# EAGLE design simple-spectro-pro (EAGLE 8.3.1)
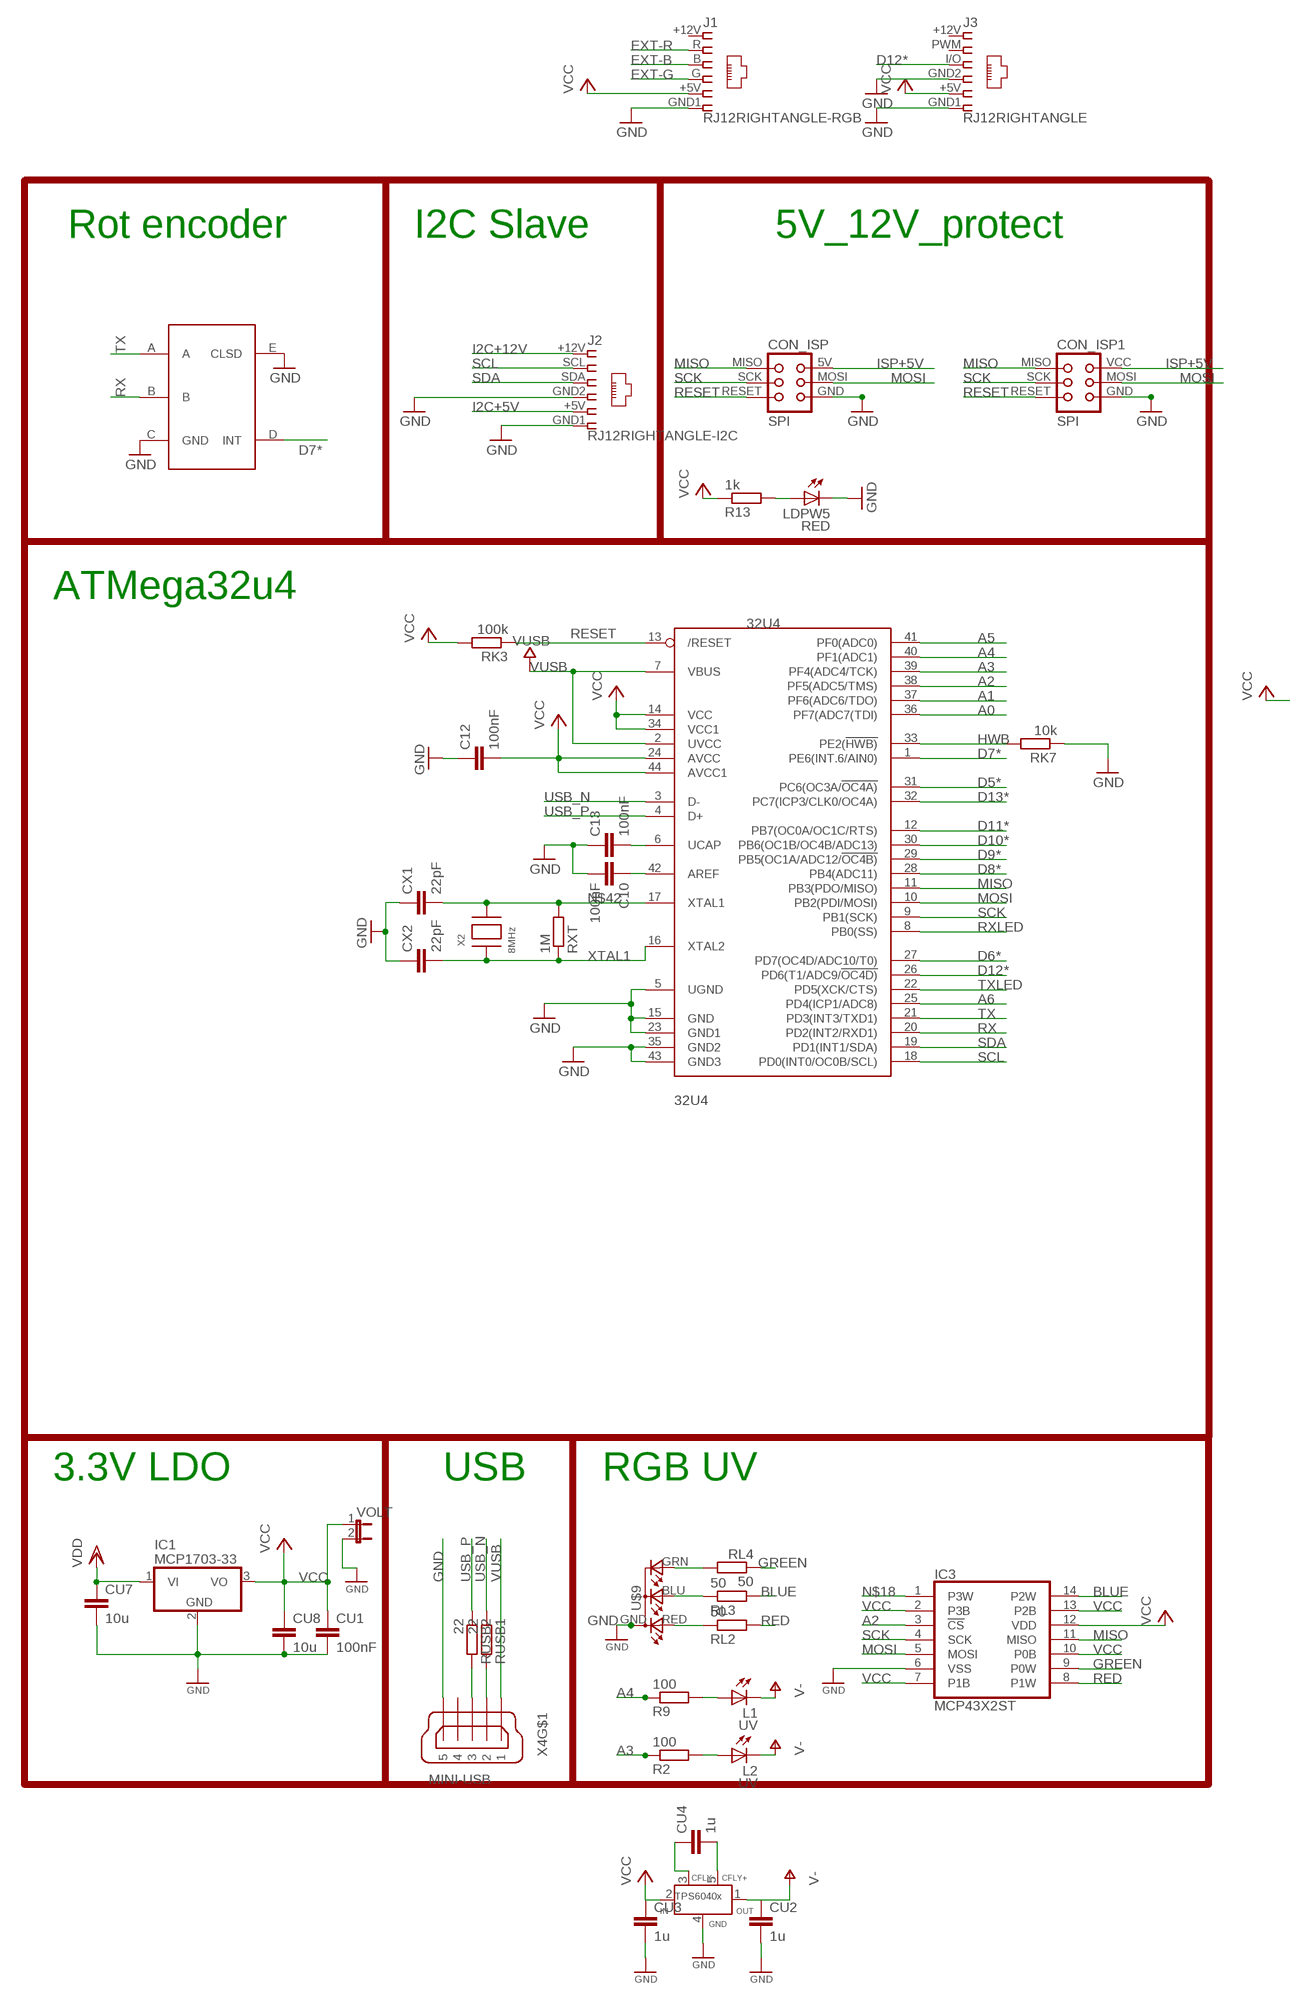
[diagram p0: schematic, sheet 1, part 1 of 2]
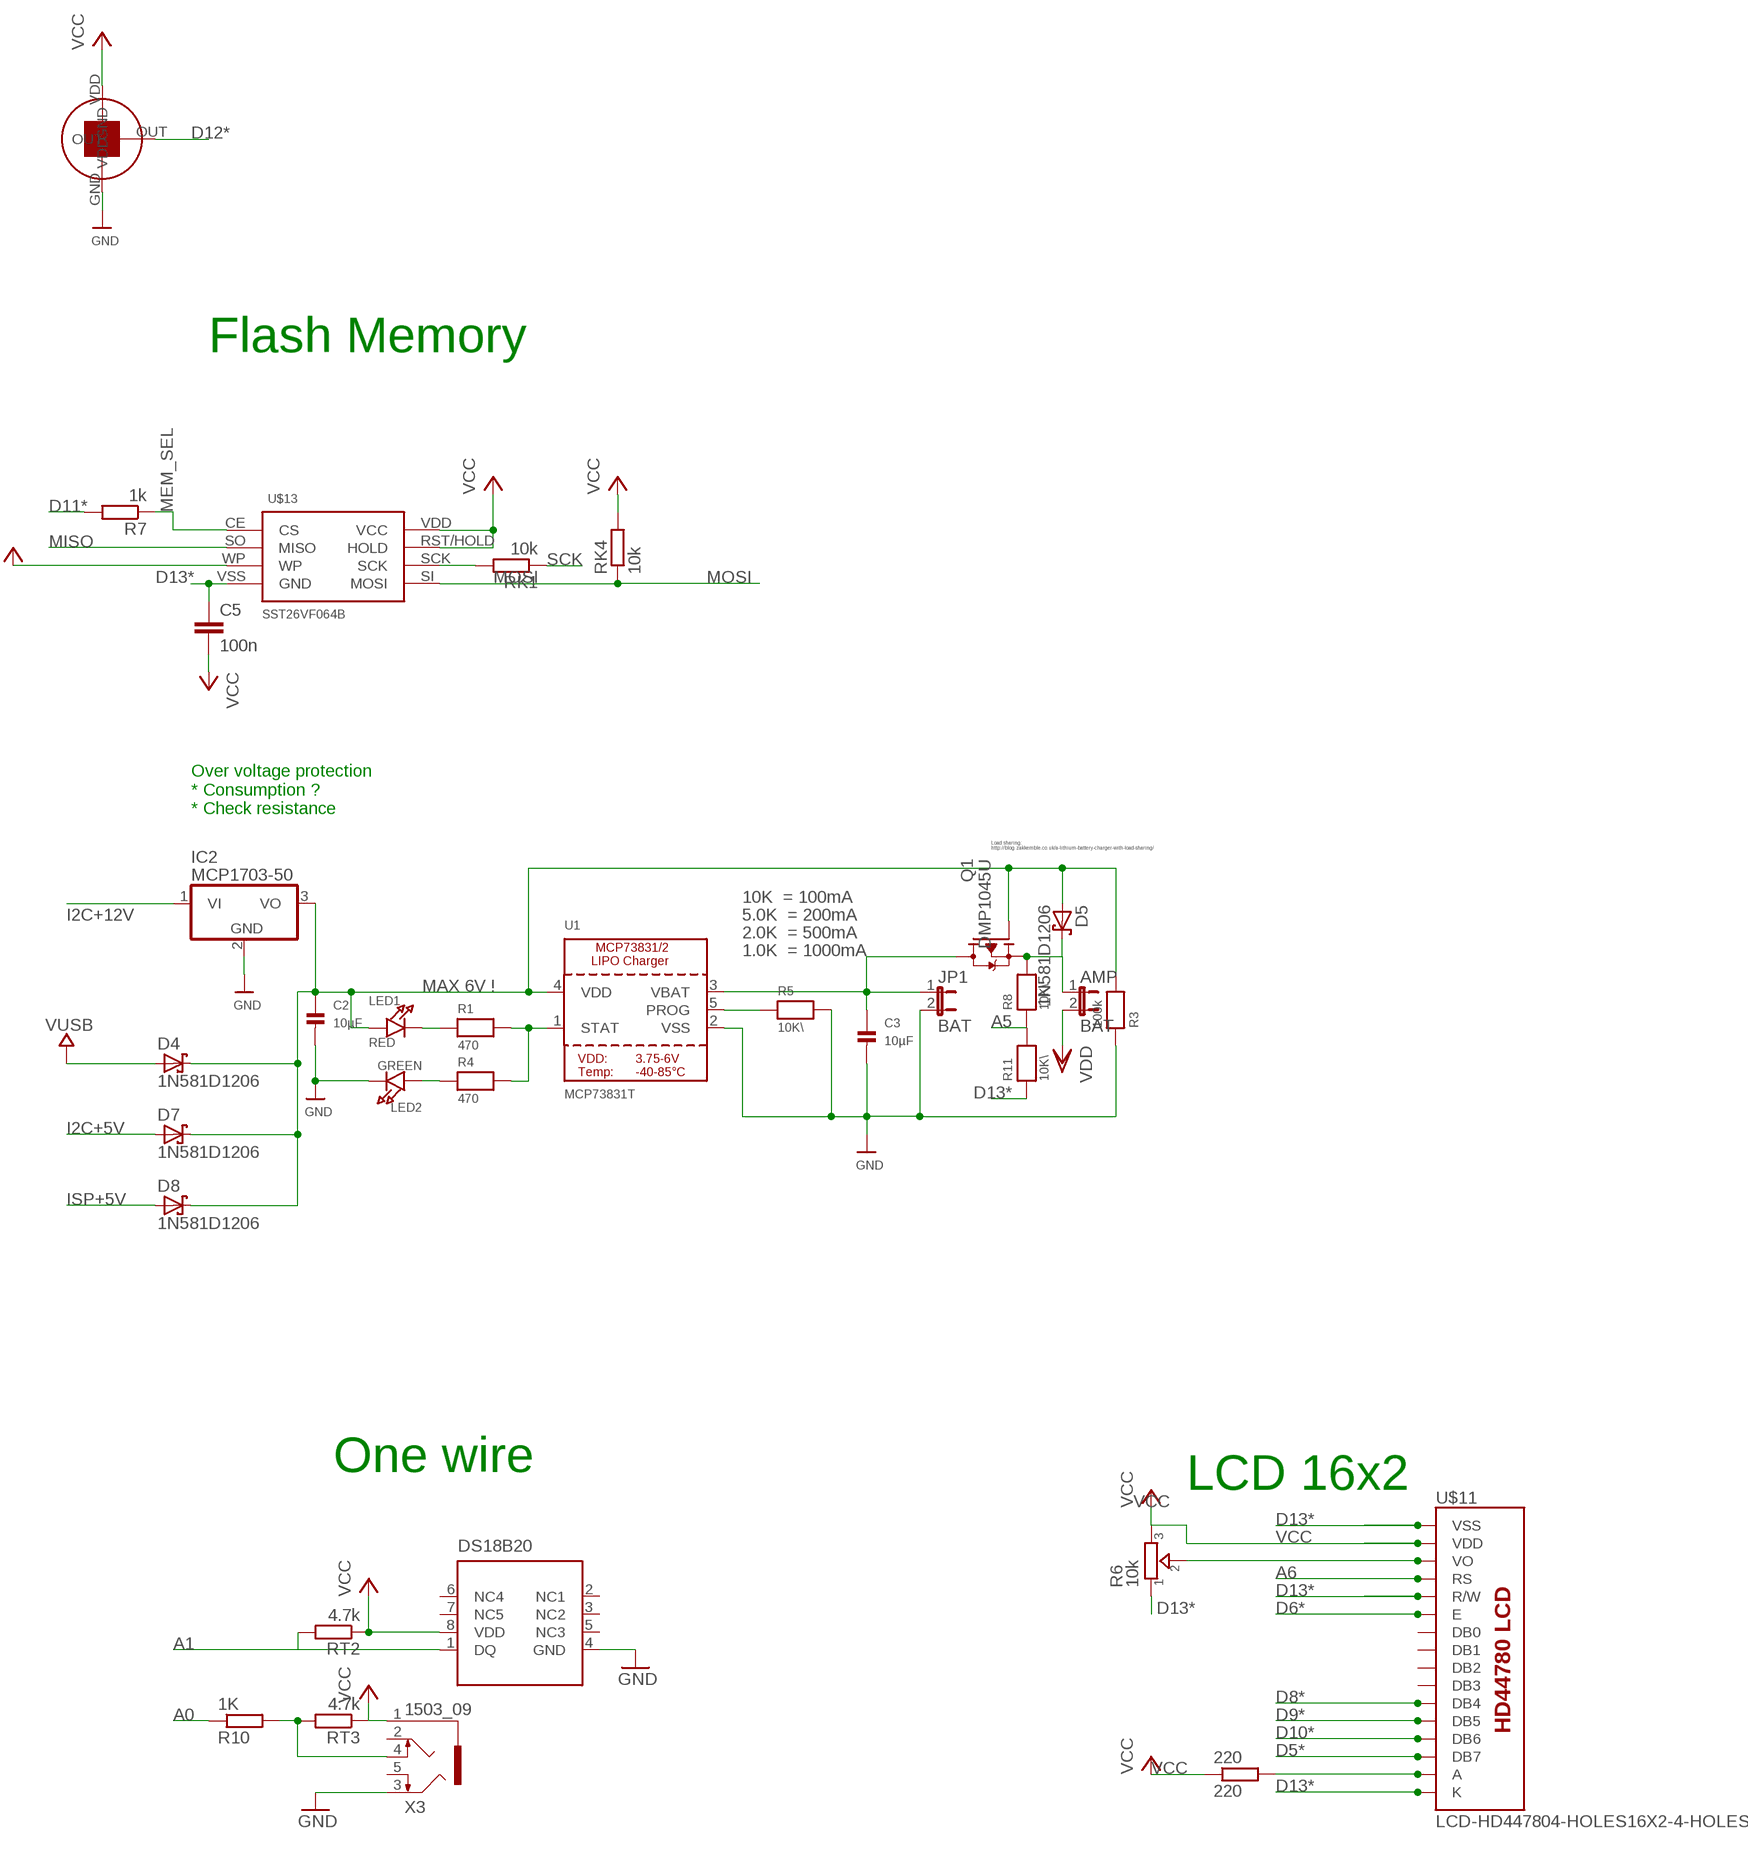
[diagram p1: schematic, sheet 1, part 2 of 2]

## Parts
32U4  32U4  ATMEGA32U4-AU  [TQFP44]
220  220  R-EU_R0805  [R0805]
AMP  BAT  JP1E  [JP1]
C2  10µF  CAP_CERAMIC0805  [0805]
C3  10µF  CAP_CERAMIC0805  [0805]
C5  100n  C-EUC0805  [C0805]
C10  100nF  C-EUC0805  [C0805]
C12  100nF  C-EUC0805  [C0805]
C13  100nF  C-EUC0805  [C0805]
CON_ISP  SPI  TINYISPT  [TC2030-MCP-NL]
CON_ISP1  SPI  TINYISP  [TINYISP]
CU1  100nF  C-EUC0805  [C0805]
CU2  1u  C-EUC0805  [C0805]
CU3  1u  C-EUC0805  [C0805]
CU4  1u  C-EUC0805  [C0805]
CU7  10u  C-EUC0805  [C0805]
CU8  10u  C-EUC0805  [C0805]
CX1  22pF  C-EUC0805  [C0805]
CX2  22pF  C-EUC0805  [C0805]
D4  1N581D1206  [LED-1206]
D5  1N581D1206  [LED-1206]
D7  1N581D1206  [LED-1206]
D8  1N581D1206  [LED-1206]
IC1  MCP1703-33  MCP1703DB  [SOT223]
IC2  MCP1703-50  MCP1703DB  [SOT223]
IC3  MCP43X2ST  [TSSOP14]
J1  RJ12RIGHTANGLE-RGB  [RJ12-RIGHTRANGE-RGB]
J2  RJ12RIGHTANGLE-I2C  [RJ12-RIGHTANGLE-I2C]
J3  RJ12RIGHTANGLE  [RJ12-RIGHTANGLE]
JP1  BAT  JP1E  [JP1]
L1  UV  LED5MM  [LED5MM]
L2  UV  LED3MM  [LED3MM]
LDPW5  RED  LEDCHIP-LED0805  [CHIP-LED0805]
LED1  RED  LED0805  [CHIPLED_0805]
LED2  GREEN  LED0805  [CHIPLED_0805]
Q1  DMP1045U  TRANSISTOR_FET_TSM2301CX  [SOT-23]
R1  470  RESISTOR0805  [0805]
R2  100  R-EU_R0805  [R0805]
R3  100k  RESISTOR0805  [0805]
R4  470  RESISTOR0805  [0805]
R5  10K\  RESISTOR0805  [0805]
R6  10k  TRIMMER-3362P  [TRIMMER_3362P]
R7  1k  R-EU_R0805  [R0805]
R8  10K\  RESISTOR0805  [0805]
R9  100  R-EU_R0805  [R0805]
R10  1K  R-EU_R0805  [R0805]
R11  10K\  RESISTOR0805  [0805]
R13  1k  R-EU_R0805  [R0805]
RK1  10k  R-EU_R0805  [R0805]
RK3  100k  R-EU_M0805  [M0805]
RK4  10k  R-EU_R0805  [R0805]
RK7  10k  R-EU_M0805  [M0805]
RL2  50  R-EU_R0805  [R0805]
RL3  50  R-EU_R0805  [R0805]
RL4  50  R-EU_R0805  [R0805]
RT2  4.7k  R-EU_R0805  [R0805]
RT3  4.7k  R-EU_R0805  [R0805]
RUSB1  22  R-EU_M0805  [M0805]
RUSB2  22  R-EU_M0805  [M0805]
RXT  1M  R-EU_R0805  [R0805]
U1  MCP73831T  MCP73831/2  [SOT23-5]
U$1  EC11E  [EC11E]
U$6  TPS6040X  [SOT23-5]
U$7  TSL237  [TSL237]
U$9  RGB-COMMON-CATHODE  [LED-TRICOLOR-THROUGHHOLE]
U$11  LCD-HD447804-HOLES16X2-4-HOLES  [LCD-16X2-4HOLES]
U$12  DS18B20  DS18B20SMALL  [MSOP8]
U$13  SST26VF064B  SST25VF064C  [SOIC_8-LEAD]
VOLT  JP1E  [JP1]
X2  8MHz  XTALNX6035  [NX6035]
X3  1503_09  [1503_09]
X4  MINI-USB  MINI-USB-SCHIELD-32005-201  [32005-201]

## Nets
A0: 32U4.36(PF7(ADC7(TDI)) R10.1
A1 [fine]: 32U4.37(PF6(ADC6/TDO)) RT2.2 U$12.1(DQ)
A2: 32U4.38(PF5(ADC5/TMS)) IC3.3(!CS)
A3: 32U4.39(PF4(ADC4/TCK)) R2.1
A4: 32U4.40(PF1(ADC1)) R9.1
A5: 32U4.41(PF0(ADC0)) R8.1 R11.2
A6: 32U4.25(PD4(ICP1/ADC8)) U$11.4(RS)
AREF: 32U4.42(AREF) C10.1
BLUE: IC3.14(P2W) RL3.2
D5*: 32U4.31(PC6(OC3A/!OC4A)) U$11.14(DB7)
D6*: 32U4.27(PD7(OC4D/ADC10/T0)) U$11.6(E)
D7*: 32U4.1(PE6(INT.6/AIN0)) U$1.D(INT)
D8*: 32U4.28(PB4(ADC11)) U$11.11(DB4)
D9*: 32U4.29(PB5(OC1A/ADC12/!OC4B)) U$11.12(DB5)
D10*: 32U4.30(PB6(OC1B/OC4B/ADC13)) U$11.13(DB6)
D11*: 32U4.12(PB7(OC0A/OC1C/RTS)) R7.2
D12*: 32U4.26(PD6(T1/ADC9/!OC4D)) J3.I/O U$7.OUT
D13*: 32U4.32(PC7(ICP3/CLK0/OC4A)) C5.1 R6.1 R11.1 U$11.1(VSS) U$11.5(R/W) U$11.16(K) U$13.VSS(GND)
EXT-B: J1.B RL3.1 U$9.BLU(CBLUE)
EXT-G: J1.G RL4.2 U$9.GRN(CGREEN)
EXT-R: J1.R RL2.1 U$9.RED(CRED)
GND [power]: 32U4.5(UGND) 32U4.15(GND) 32U4.23(GND1) 32U4.35(GND2) 32U4.43(GND3) C2.2 C3.2 C10.2 C12.1 C13.1 CON_ISP1.GND CON_ISP.GND CU1.2 CU2.2 CU3.2 CU7.2 CU8.2 CX1.1 CX2.1 IC1.2(GND) IC2.2(GND) IC3.6(VSS) J1.GND1 J2.GND1 J2.GND2 J3.GND1 J3.GND2 JP1.2 LDPW5.C LED2.C R3.1 R5.2 RK7.1 U1.2(VSS) U$1.C(GND) U$1.E(CLSD) U$6.4(GND) U$7.GND U$9.GND(A2) U$12.4(GND) VOLT.2 X3.3 X4.5
GREEN: IC3.9(P0W) RL4.1
HWB: 32U4.33(PE2(!HWB)) RK7.2
I2C+5V: D7.A J2.+5V
I2C+12V [power]: IC2.1(VI) J2.+12V
ISP+5V: CON_ISP1.VCC CON_ISP.5V(VCC) D8.A
MEM_SEL: R7.1 U$13.CE(CS)
MISO: 32U4.11(PB3(PDO/MISO)) CON_ISP1.MISO CON_ISP.MISO IC3.11(MISO) U$13.SO(MISO)
MOSI: 32U4.10(PB2(PDI/MOSI)) CON_ISP1.MOSI CON_ISP.MOSI IC3.5(MOSI) RK4.1 U$13.SI(MOSI)
N$1: 32U4.6(UCAP) C13.2
N$2: R6.2 U$11.3(VO)
N$3: L1.A R9.2
N$4: LED1.C R1.1
N$5: R1.2 R4.2 U1.1(STAT)
N$6: R5.1 U1.5(PROG)
N$7: LED2.A R4.1
N$8: L2.A R2.2
N$9 [power]: R10.2 RT3.2 X3.4
N$11: 220.2 U$11.15(A)
N$12: LDPW5.A R13.2
N$15: C2.1 D4.C D5.A D7.C D8.C IC2.3(VO) LED1.A Q1.1(G) R3.2 U1.4(VDD)
N$17 [power]: AMP.1 D5.C Q1.2(S) R8.2
N$18: IC3.1(P3W)
N$19: CU4.2 U$6.5(CFLY+)
N$20: CU4.1 U$6.3(CFLY-)
N$23: RK1.2 U$13.SCK
N$42: 32U4.17(XTAL1) CX1.2 RXT.2 X2.P$2
RED: IC3.8(P1W) RL2.2
RESET: 32U4.13(/RESET) CON_ISP1.RESET CON_ISP.RESET RK3.1
RX: 32U4.20(PD2(INT2/RXD1)) U$1.B
RXLED: 32U4.8(PB0(SS))
SCK: 32U4.9(PB1(SCK)) CON_ISP1.SCK CON_ISP.SCK IC3.4(SCK) RK1.1
SCL: 32U4.18(PD0(INT0/OC0B/SCL)) J2.SCL
SDA: 32U4.19(PD1(INT1/SDA)) J2.SDA
TX: 32U4.21(PD3(INT3/TXD1)) U$1.A
TXLED: 32U4.22(PD5(XCK/CTS))
USB_N: 32U4.3(D-) RUSB1.1
USB_P: 32U4.4(D+) RUSB2.1
USBC_N: RUSB1.2 X4.2
USBC_P: RUSB2.2 X4.3
V- [power]: CU2.1 L1.K(C) L2.K(C) U$6.1(OUT)
VBAT1: C3.1 JP1.1 Q1.3(D) U1.3(VBAT)
VCC: 32U4.14(VCC) 32U4.24(AVCC) 32U4.34(VCC1) 32U4.44(AVCC1) 220.1 C5.2 C12.2 CU1.1 CU3.1 CU8.1 IC1.3(VO) IC3.2(P3B) IC3.7(P1B) IC3.10(P0B) IC3.12(VDD) IC3.13(P2B) J1.+5V J3.+5V R6.3 R13.1 RK3.2 RK4.2 RT2.1 RT3.1 U$6.2(IN) U$7.VDD U$11.2(VDD) U$12.8(VDD) U$13.RST/HOLD(HOLD) U$13.VDD(VCC) U$13.WP VOLT.1 X3.1
VDD [power]: AMP.2 CU7.1 IC1.1(VI)
VUSB: 32U4.2(UVCC) 32U4.7(VBUS) D4.A X4.1
XTAL1: 32U4.16(XTAL2) CX2.2 RXT.1 X2.P$1
Unconnected: J1.+12V J3.+12V J3.PWM U$11.7(DB0) U$11.8(DB1) U$11.9(DB2) U$11.10(DB3) U$12.2(NC1) U$12.3(NC2) U$12.5(NC3) U$12.6(NC4) U$12.7(NC5) X3.2 X3.5 X4.4 X4.M1(S:S1) X4.M2(S:S2) X4.M3(S:S3) X4.M4(S:S4)

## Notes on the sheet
- Rot encoder | I2C Slave | 5V_12V_protect
- Flash Memory
- ATMega32u4
- Over voltage protection
  * Consumption ?
  * Check resistance
- Load sharing:
  http://blog.zakkemble.co.uk/a-lithium-battery-charger-with-load-sharing/
- 10K  = 100mA
- 5.0K  = 200mA
- 2.0K  = 500mA
- 1.0K  = 1000mA
- MAX 6V !
- One wire
- LCD 16x2
- 3.3V LDO | USB | RGB UV

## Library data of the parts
32U4 = adafruit:ATMEGA32U4: http://www.ladyada.net/library/eagle
220 R2 R7 R9 R10 RK1 RK4 RL2-RL4 RXT = rcl:R-EU_: RESISTOR, European symbol
AMP JP1 VOLT = jumper:JP1E: JUMPER
C2 C3 = microbuilder:CAP_CERAMIC: Ceramic Capacitors
C5 C10 C12 C13 CU1-CU4 CU7 CU8 CX1 CX2 = rcl:C-EU: CAPACITOR, European symbol
CON_ISP = lpatiny:TINYISP: CONNECTOR
CON_ISP1 = lpatiny:TINYISP: CONNECTOR; OC_FARNELL: unknown; OC_NEWARK: unknown
D4 D5 D7 D8 = lpatiny:1N581*: 1.0A SCHOTTKY BARRIER RECTIFIER
IC1 IC2 = linear:MCP1703: 250 mA, 16V, Low Quiescent Current LDO Regulator Source: http://ww1.microchip.com/downloads/en/DeviceDoc/22049b.pdf
IC3 = microchip-mcp43x2:MCP43X2: Quad Rheostat
J1-J3 = lpatiny:RJ12: CORCOM Modular RJ Jacks No Shield Source: www.tycoelectronics.com .. ENG_DS_1654001_1099_RJ_L_0507.pdf
L1 = SparkFun:LED: LEDs
L2 = led:LED: LED
LDPW5 = adafruit:LED: LED
LED1 LED2 = microbuilder:LED: LED
Q1 = dp_devices:TRANSISTOR_FET_TSM2301CX: 20V P-Channel Enhancement Mode MOSFET
R1 R3-R5 R8 R11 = microbuilder:RESISTOR: Resistors
R6 = dp_devices:TRIMMER: Trimmer resistor
R13 RK3 RK7 RT2 RT3 RUSB1 RUSB2 = resistor:R-EU_: RESISTOR, European symbol
U1 = microbuilder:MCP73831/2: MCP73831/2 LIPO Charger VDD: 3.75 - 6V Temp -40 - 85°C Programmable Charge Rate: 15-500mA NOTE: STAT is a tri-state logic output on the MCP73831 and an open-drain output on the MCP73832. SOT23-5 with 4.2V output and tri-state logic on STAT = MCP73831T-2ACI/OT
U$1 = lpatiny:EC11E: ALPS Rotary encoder
U$6 = lpatiny:TPS6040X
U$7 = lpatiny:TSL237
U$9 = lpatiny:RGB-COMMON-CATHODE
U$11 = HD44780LCD:LCD-HD44780
U$12 = lpatiny:DS18B20
U$13 = BertaLib:SST25VF064C
X2 = lpatiny:XTAL: Low cost SMT crystals, no capacitors included
X3 = con-lumberg:1503_09: Jack connectors according to JISC 6560, 3.5 mm Klinkeneinbaukupplung nach JISC 6560, 3,5 mm, 3-polig/ stereo, abgewinkelte Ausführung, mit 2 Öffnern und Lötaugen, für Leiterplatten Rückseitenmontage Source: http://www.lumberg.com/Produkte/PDFs/1503_09.pdf; OC_FARNELL: 1243244; OC_NEWARK: unknown
X4 = con-cypressindustries:MINI-USB-SCHIELD-: MINI USB-B Conector Source: www.cypressindustries.com; OC_FARNELL: unknown; OC_NEWARK: unknown

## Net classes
0 default: width 0.406 mm, clearance 0.25 mm
1 power: width 0.406 mm, drill 0.305 mm, clearance 0.25 mm
2 VIN: width 0.406 mm, clearance 0.25 mm
3 fine: width 0.305 mm, clearance 0.25 mm
4 aref: width 0.406 mm, clearance 0.25 mm

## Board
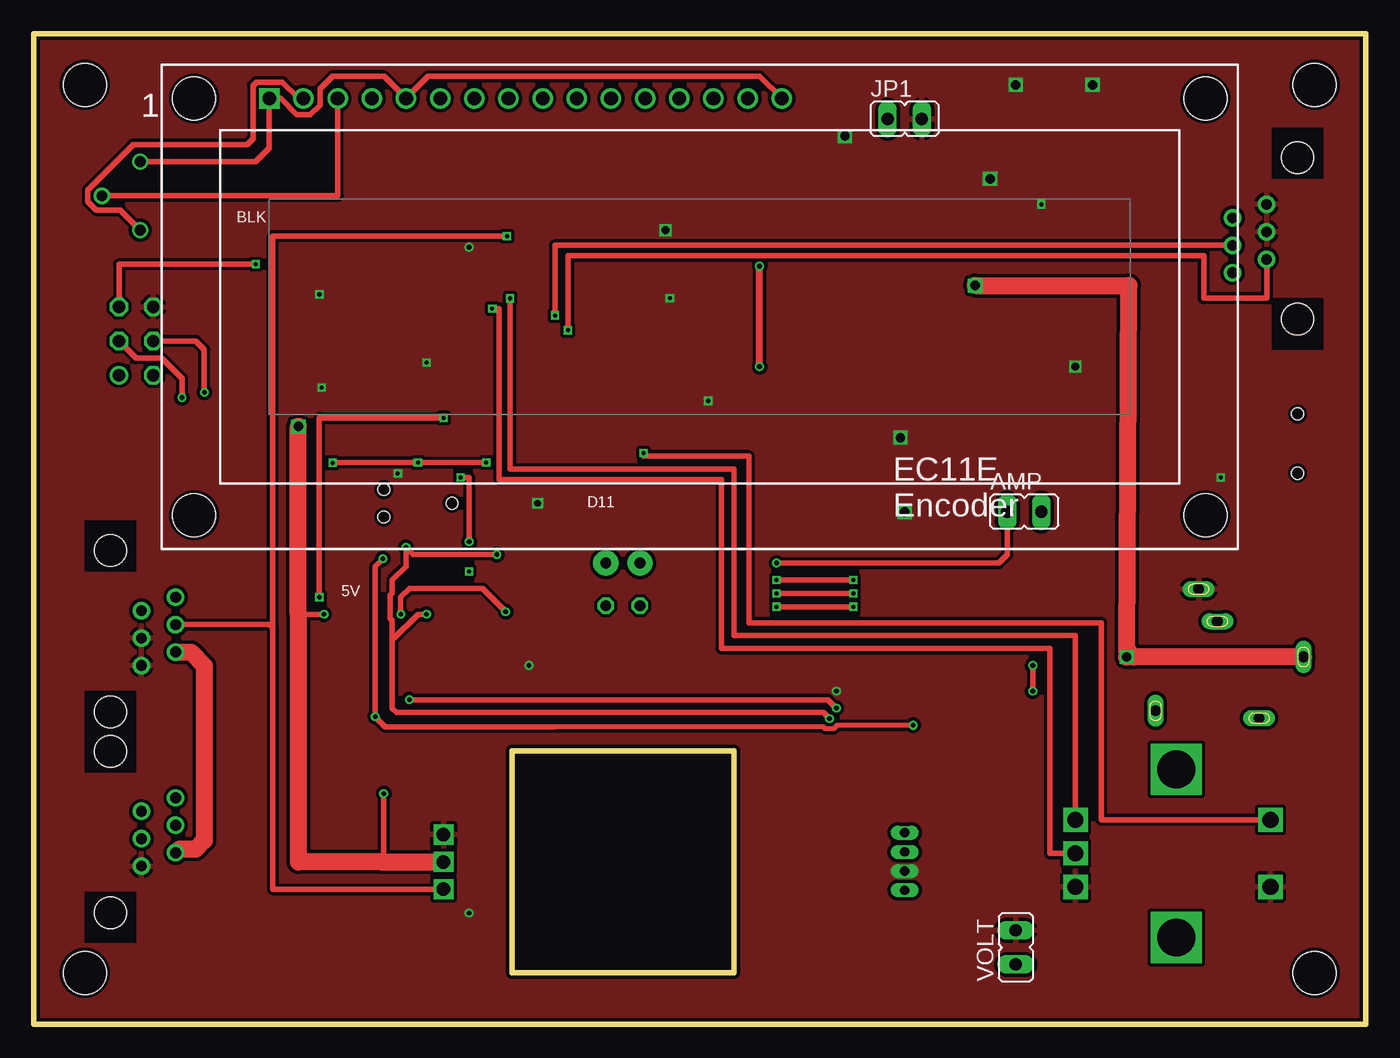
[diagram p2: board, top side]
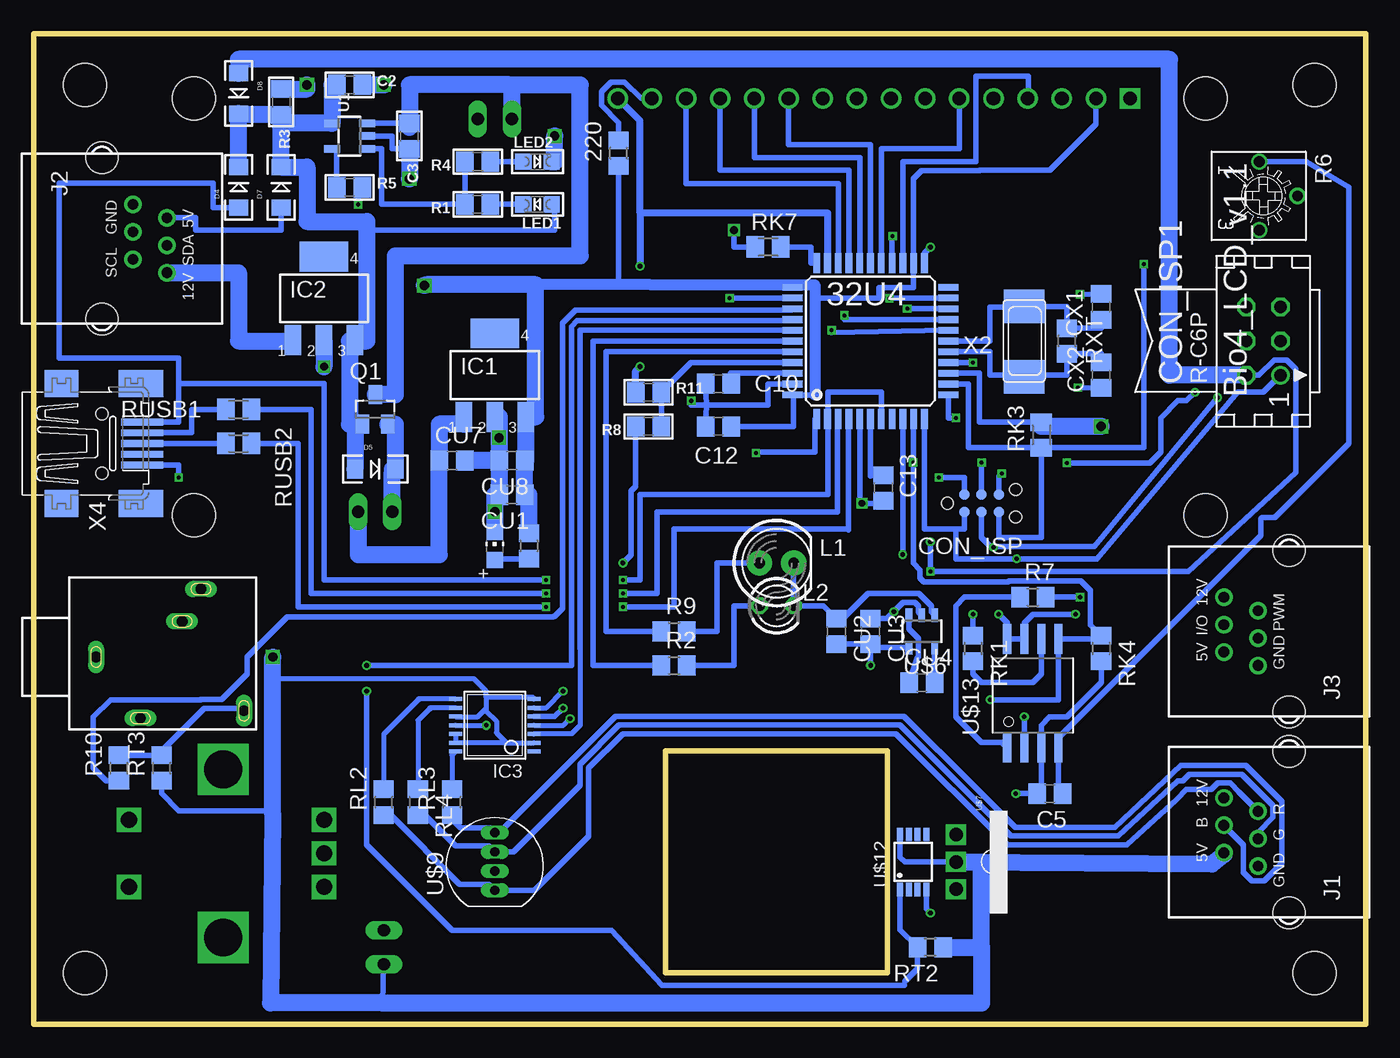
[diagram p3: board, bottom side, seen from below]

Size 99.06 x 73.66 mm. Coordinates in mm from the lower left corner, seen from the top.
Outline: 0,73.66 0,0 99.06,0 99.06,73.66 0,73.66
Outline: 35.56,20.32 52.07,20.32 52.07,3.81 35.56,3.81 35.56,20.32
Copper layers (1*2*15*16): Top 0.035mm / dielectric 0.2mm / layer 2 0.0175mm / dielectric 1.1mm / layer 15 0.0175mm / dielectric 0.2mm / Bottom 0.035mm
Design rules "SeeedStudio_DRU_no_angle_20130527": minimum track width 6mil, minimum drill 12mil, track to track 6mil, track to pad 6mil, pad to pad 6mil, via to via 6mil, smd to smd 0mil, copper to edge 10mil, drill to drill 10mil, minimum pad ring 6mil, minimum via ring 6mil, stop-mask expansion 2mil, vias tented up to drill 25mil, thermal gap 10mil
Holes 3.2 mm at 3.81,69.85 3.81,3.81 95.25,69.85 95.25,3.81

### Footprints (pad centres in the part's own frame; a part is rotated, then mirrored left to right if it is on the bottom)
TQFP44 = smd 1.5 x 0.5: 1 -5.8,4; 2 -5.8,3.2; 3 -5.8,2.4; 4 -5.8,1.6; 5 -5.8,0.8; 6 -5.8,0; 7 -5.8,-0.8; 8 -5.8,-1.6; 9 -5.8,-2.4; 10 -5.8,-3.2; 11 -5.8,-4; 23 5.8,-4; 24 5.8,-3.2; 25 5.8,-2.4; 26 5.8,-1.6; 27 5.8,-0.8; 28 5.8,0; 29 5.8,0.8; 30 5.8,1.6; 31 5.8,2.4; 32 5.8,3.2; 33 5.8,4 | smd 0.5 x 1.5: 12 -4,-5.8; 13 -3.2,-5.8; 14 -2.4,-5.8; 15 -1.6,-5.8; 16 -0.8,-5.8; 17 0,-5.8; 18 0.8,-5.8; 19 1.6,-5.8; 20 2.4,-5.8; 21 3.2,-5.8; 22 4,-5.8; 34 4,5.8; 35 3.2,5.8; 36 2.4,5.8; 37 1.6,5.8; 38 0.8,5.8; 39 0,5.8; 40 -0.8,5.8; 41 -1.6,5.8; 42 -2.4,5.8; 43 -3.2,5.8; 44 -4,5.8
R0805 = smd 1.3 x 1.5: 1 -0.95,0; 2 0.95,0
JP1 = drill 0.914 long: 1 0,-1.27; 2 0,1.27
0805 = smd 1.3 x 1.5: 1 -0.95,0; 2 0.95,0
C0805 = smd 1.3 x 1.5: 1 -0.95,0; 2 0.95,0
TC2030-MCP-NL = smd 0.787 x 0.787: 5V 1.27,0.635; GND 3.81,0.635; MISO 1.27,-0.635; MOSI 2.54,0.635; RESET 3.81,-0.635; SCK 2.54,-0.635 | hole 0.889: 0,0; 5.08,-1.016; 5.08,1.016
TINYISP = drill 0.914 octagon: GND 2.54,1.27; MOSI 0,1.27; RESET 2.54,-1.27; SCK 0,-1.27; VCC -2.54,1.27 | drill 0.914: MISO -2.54,-1.27
LED-1206 = smd 1.2 x 1.4: A -1.5,0; C 1.5,0
SOT223 = smd 1.219 x 2.235: 1 -2.311,-3.099; 2 0,-3.099; 3 2.311,-3.099 | smd 3.6 x 2.2: 4 0,3.099
TSSOP14 = smd 0.305 x 0.991: 1 -1.95,-2.918; 2 -1.3,-2.918; 3 -0.65,-2.918; 4 0,-2.918; 5 0.65,-2.918; 6 1.3,-2.918; 7 1.95,-2.918; 8 1.95,2.918; 9 1.3,2.918; 10 0.65,2.918; 11 0,2.918; 12 -0.65,2.918; 13 -1.3,2.918; 14 -1.95,2.918
RJ12-RIGHTRANGE-RGB = drill 0.8 pad 1.3: +5V -1.54,4.84; +12V 2.54,4.84; B 0.5,4.84; G -0.5,2.3; GND1 -2.54,2.3; R 1.54,2.3 | hole 2.36: -6,0; 6,0
RJ12-RIGHTANGLE-I2C = drill 0.8 pad 1.3: +5V -1.54,4.84; +12V 2.54,4.84; GND1 -2.54,2.3; GND2 -0.5,2.3; SCL 1.54,2.3; SDA 0.5,4.84 | hole 2.36: -6,0; 6,0
RJ12-RIGHTANGLE = drill 0.8 pad 1.3: +5V -1.54,4.84; +12V 2.54,4.84; GND1 -2.54,2.3; GND2 -0.5,2.3; I/O 0.5,4.84; PWM 1.54,2.3 | hole 2.36: -6,0; 6,0
LED5MM = drill 0.813 pad 1.88: A -1.27,0; K 1.27,0
LED3MM = drill 0.813 octagon: A -1.27,0; K 1.27,0
CHIP-LED0805 = smd 1.2 x 1.2: A 0,-1.05; C 0,1.05
CHIPLED_0805 = smd 1.2 x 1.2: A 0,-1.05; C 0,1.05
SOT-23 = smd 1 x 1.4: 1 -0.95,-1.1; 2 0.95,-1.1; 3 0,1.1
TRIMMER_3362P = drill 0.8: 1 -2.54,-0.31; 2 0,2.54; 3 2.54,-0.31
M0805 = smd 1.3 x 1.6: 1 -0.95,0; 2 0.95,0
SOT23-5 = smd 0.55 x 1.2: 1 -0.95,-1.3; 2 0,-1.3; 3 0.95,-1.3; 4 0.95,1.3; 5 -0.95,1.3
EC11E = drill 1.2 square: A -2.5,0; B 0,0; C 2.5,0; D -2.5,14.5; E 2.5,14.5 | drill 2.8 square: P$1 6.25,7.5; P$2 -6.25,7.5
SOT23-5' = smd 0.5 x 1: 1 -0.95,-1.2; 2 0,-1.2; 3 0.95,-1.2; 4 0.95,1.2; 5 -0.95,1.2
TSL237 = drill 1 pad 1.27 square: GND -2.032,-2.54; OUT 2.032,-2.54; VDD 0,-2.54
LED-TRICOLOR-THROUGHHOLE = drill 0.7 long: BLU 2.175,0; GND -0.682,0; GRN 0.746,0; RED -2.111,0
LCD-16X2-4HOLES = drill 1.016 square: 1 -32,15.5 | drill 1.016: 2 -29.46,15.5; 3 -26.92,15.5; 4 -24.38,15.5; 5 -21.84,15.5; 6 -19.3,15.5; 7 -16.76,15.5; 8 -14.22,15.5; 9 -11.68,15.5; 10 -9.14,15.5; 11 -6.6,15.5; 12 -4.06,15.5; 13 -1.52,15.5; 14 1.02,15.5; 15 3.56,15.5; 16 6.1,15.5 | hole 3.2: -37.6,15.5; -37.6,-15.5; 37.6,-15.5; 37.6,15.5
MSOP8 = smd 0.45 x 1: 1 -0.975,-2.05; 2 -0.325,-2.05; 3 0.325,-2.05; 4 0.975,-2.05; 5 0.975,2.05; 6 0.325,2.05; 7 -0.325,2.05; 8 -0.975,2.05
SOIC_8-LEAD = smd 0.61 x 2.21: CE -1.905,-2.934; RST/HOLD -0.635,5.156; SCK 0.635,5.156; SI 1.905,5.156; SO -0.635,-2.934; VDD -1.905,5.156; VSS 1.905,-2.934; WP 0.635,-2.934
NX6035 = smd 2.5 x 3: P$1 2.665,0; P$2 -2.565,0
1503_09 = drill 0.8 pad 1.2 long: 1 0,-2.1; 2 -4.55,-5.4; 3 5.05,-9.9; 4 -4,-13.1; 5 2.65,-8.5
32005-201 = smd 3.1 x 0.5: 1 3,1.6; 2 3,0.8; 3 3,0; 4 3,-0.8; 5 3,-1.6 | smd 2.5 x 2: M1 -3,-4.45; M2 -3,4.45 | smd 3.3 x 2: M3 2.9,4.45; M4 2.9,-4.45 | hole 0.9: 0,2.2; 0,-2.2

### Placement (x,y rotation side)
32U4  36.83,50.8 90 bottom
220  55.56,64.77 90 bottom
AMP  73.66,38.1 270 top
C2  75.56,69.85 0 bottom
C3  71.12,66.04 270 bottom
C5  23.5,17.14 180 bottom
C10  48.14,47.62 180 bottom
C12  48.14,44.45 0 bottom
C13  35.88,39.88 90 bottom
CON_ISP  31.11,38.73 0 bottom
CON_ISP1  7.62,50.8 90 bottom
CU1  63.5,39.37 180 bottom
CU2  39.37,29.21 270 bottom
CU3  36.83,29.21 270 bottom
CU4  33.02,25.4 0 bottom
CU7  67.94,41.91 0 bottom
CU8  63.5,41.91 180 bottom
CX1  19.68,53.34 270 bottom
CX2  19.68,48.26 90 bottom
D4  83.82,62.23 90 bottom
D5  73.66,41.27 0 bottom
D7  80.64,62.23 90 bottom
D8  83.82,69.22 270 bottom
IC1  64.77,48.26 0 bottom
IC2  77.47,53.98 0 bottom
IC3  64.77,22.23 90 bottom
J1  5.71,14.29 90 bottom
J2  93.98,58.42 270 bottom
J3  5.71,29.21 90 bottom
JP1  64.77,67.31 270 top
L1  43.81,34.29 0 bottom
L2  43.81,31.11 0 bottom
LDPW5  64.77,35.56 0 bottom
LED1  61.59,60.96 90 bottom
LED2  61.59,64.14 270 bottom
Q1  73.66,45.72 0 bottom
R1  66.04,60.96 180 bottom
R2  51.44,26.67 0 bottom
R3  80.64,68.58 270 bottom
R4  66.04,64.14 180 bottom
R5  75.56,62.23 0 bottom
R6  7.62,61.59 270 bottom
R7  24.77,31.75 0 bottom
R8  53.34,44.45 180 bottom
R9  51.44,29.21 0 bottom
R10  92.71,19.05 90 bottom
R11  53.34,46.99 0 bottom
R13  62.23,35.56 270 bottom
RK1  29.21,27.94 270 bottom
RK3  24.13,43.81 90 bottom
RK4  19.68,27.94 270 bottom
RK7  44.45,57.78 0 bottom
RL2  73.03,16.51 90 bottom
RL3  67.94,16.51 90 bottom
RL4  70.48,16.51 270 bottom
RT2  32.38,5.71 180 bottom
RT3  89.53,19.05 90 bottom
RUSB1  83.82,45.72 180 bottom
RUSB2  83.82,43.18 180 bottom
RXT  22.23,50.8 90 bottom
U1  75.56,66.04 90 bottom
U$1  77.47,12.7 270 top
U$6  TPS6040X  [SOT23-5']  33.02,29.21 180 bottom
U$7  27.94,12.06 270 bottom
U$9  64.77,12.06 90 bottom
U$11  49.53,53.34 0 top
U$12  33.66,12.06 0 bottom
U$13  24.77,23.5 0 bottom
VOLT  73.03,5.71 0 top
X2  25.4,50.8 270 bottom
X3  96.52,27.3 90 bottom
X4  93.98,43.18 0 bottom

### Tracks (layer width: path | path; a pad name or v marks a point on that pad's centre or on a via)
A0
  Bottom 0.406: R10.1 93.67,18.1 94.61,19.05 94.61,22.86 93.34,24.13 86.65,24.13 86.63,24.15 85.07,24.15 83.19,26.04 83.19,27.3 80.21,30.28 60.45,30.28 60.41,30.32 60.33,30.32 59.73,30.91 59.73,52.14 58.77,53.1 42.73,53.1 32U4.36
A1  (via drill 0.35)
  Top 0.406: v74.3,26.67 v74.3,24.77
  Bottom 0.305: 33.36,5.74 RT2.2 | 34.31,2.88 34.29,3.17
  Bottom 0.406: 32U4.37 42.73,52.3 58.65,52.3 59.08,51.87 59.08,27.67 59.05,27.65 59.05,26.67 v74.3,26.67 | v74.3,24.77 74.3,13.34 67.94,6.99 56.11,6.99 52.32,2.88 34.31,2.88 | U$12.1 34.63,7.01 33.36,5.74 33.36,4.11 34.29,3.17
A2
  Bottom 0.356: 58.42,27.94 58.42,22.23 59.05,21.59 61.84,21.59 IC3.3
  Bottom 0.406: 32U4.38 58.42,51.6 58.42,27.94
A3
  Bottom 0.406: 32U4.39 57.48,50.8 57.48,26.67 R2.1
A4
  Bottom 0.406: 42.63,50.04 32U4.40 56.52,50 56.52,29.21 R9.1
A5
  Bottom 0.406: 42.63,49.21 32U4.41 50.18,49.2 R11.2 R8.1
A6
  Bottom 0.406: U$11.4 25.08,68.84 25.08,70.48 29,70.48 29,64.14 34.43,64.14 32U4.25
AREF
  Bottom 0.406: 32U4.42 47.25,48.4 C10.1
BLUE
  Bottom 0.356: IC3.14 67.94,20.02 RL3.2
  Bottom 0.406: RL3.2 67.94,17.48
D5*
  Bottom 0.406: 39.24,56.6 32U4.31 39.23,62.5 50.55,62.5 U$11.14
D6*
  Bottom 0.406: 32U4.27 36.03,65.09 30.23,65.09 U$11.6
D7*  (via drill 0.3)
  Top 0.406: U$1.D 79.38,15.2 79.38,29.84 53.17,29.84 53.17,42.24 45.34,42.24 v45.34,42.48
  Bottom 0.406: 32U4.1 40.96,45 40.96,42.55 45.34,42.55 v45.34,42.48 | 91.97,14.93 U$1.D
D8*
  Bottom 0.406: 32U4.28 36.83,65.41 42.93,65.41 U$11.11
D9*
  Bottom 0.406: 32U4.29 37.63,64.45 45.47,64.45 U$11.12
D10*
  Bottom 0.406: 32U4.30 38.43,63.5 48.01,63.5 U$11.13
D11*  (via drill 0.3)
  Top 0.406: v21.25,31.75 21.25,45.09 v30.48,45.09
  Bottom 0.406: v30.48,45.09 31.03,45.09 32U4.12 | v21.25,31.75 R7.2
D12*  (via drill 0.3)
  Top 0.406: v35.19,58.61 17.78,58.61 17.78,29.5 | 17.78,29.5 17.78,10.03 U$7.OUT | J3.I/O 17.57,29.71 17.78,29.5
  Bottom 0.406: 32U4.26 35.24,58.51 35.19,58.51 v35.19,58.61
D13*  (via drill 0.35)
  Top 0.406: R6.1 16.51,64.14 17.53,65.16 U$11.1 18.35,68.84 19.57,67.62 20.57,67.62 21.29,68.34 21.29,69.55 22.23,70.48 26.05,70.48 U$11.5 29.34,70.48 53.98,70.48 U$11.16
  Top 0.508: v53.98,48.9 v53.98,56.37
  Bottom 0.406: 32U4.32 40.01,56.6 | 53.95,60.33 53.98,60.35 | C5.1 22.86,17.46 U$13.VSS 22.86,21.3 7.82,36.33 7.82,37.55 7.7,37.67 6.78,37.67 1.27,43.18 1.27,62.23 4.45,64.14 R6.1
  Bottom 0.508: 40.01,56.6 40.01,60.33 53.95,60.33 | R11.1 54.29,48.58 v53.98,48.9 | v53.98,56.37 53.98,60.35 53.98,67.19 U$11.16
EXT-B
  Bottom 0.406: RL3.1 67.94,15.24 67.31,14.61 65.14,14.61 U$9.BLU 64.45,14.24 55.79,22.9 34.65,22.9 | 34.65,22.9 34.38,22.9 | J1.B 9.12,13.35 9.12,11.29 8.47,10.64 7.56,10.64 6.25,11.95 6.25,16.56 8.94,19.24 13.75,19.24 18.66,14.65 26.08,14.65 29.21,17.78 | 29.38,17.95 29.21,17.78 | 29.21,17.78 34.33,22.9 34.65,22.9
EXT-G
  Bottom 0.406: RL4.2 69.99,15.56 67.69,13.26 65.22,13.26 U$9.GRN 63.39,12.81 58.44,17.76 58.44,19.32 55.52,22.25 34.65,22.25 26.4,13.99 18.39,13.99 13.97,18.1 13.63,18.1 13.14,18.59 9.21,18.59 6.91,16.28 6.91,15.37 8.02,14.27 J1.G
EXT-R
  Bottom 0.406: RL2.1 72.53,15.56 67.37,10.4 65.22,10.4 U$9.RED 61.8,9.95 57.78,13.97 57.78,19.05 55.24,21.59 34.97,21.59 | 34.97,21.59 34.92,21.59 | 14.07,16.73 14.61,16.19 | 14.07,16.73 13.34,17.46 11.48,17.46 11.01,17.93 10.1,17.93 9.45,17.28 9.45,17.26 J1.R | 14.07,16.73 17.78,13.34 26.67,13.34 34.92,21.59 | 34.92,21.59 34.97,21.59
GND  (via drill 0.3, 0.35, 0.5 pad 0.61, 0.6, 0.7)
  Bottom 0.356: IC3.6 60.93,23.52 v59.69,24.77
  Bottom 0.406: 49.02,47.6 C10.2 49.02,46.04 | 49.02,46.04 C12.1 | 32U4.43 44.45,47.6 44.45,46.04 49.02,46.04 | v50.16,46.35 50.16,46.04 49.02,46.04 | 32U4.5 37.63,38.73 v37.47,38.73 35.88,38.73 C13.1 | C3.2 72.39,65.09 72.39,66.04 U1.2 | 64.77,41.91 CU8.2 | CU1.2 64.77,39.37 | X4.5 88.27,41.58 v88.27,40.64 | 32U4.35 v47.3,54 | CX1.1 v21.25,54.27 | 32U4.15 v29.22,49.2 | v29.22,49.2 | 32.85,56.6 32U4.23 32.83,57.34 v32.38,57.78 | CON_ISP.GND 27.3,40.72 v27.08,40.95 | RK7.1 46.99,57.78 v46.99,59.05 | CX2.1 v21.42,47.33 | R5.2 74.93,62.23 v74.93,60.96 | U$6.4 36.58,28.01 CU3.2 | CU2.2 CU3.2 | U$12.4 32.68,8.6 v32.38,8.26 | CU3.2 v36.83,26.67
  Bottom 1.27: IC2.2 v77.47,48.9 | LED2.C 60.33,64.14 v60.33,66.04 | C3.2 v71.12,62.87 | C2.2 v73.03,69.85 | R3.1 78.74,69.53 v78.74,69.85 | IC1.2 64.45,45.16 v64.45,43.62 CU8.2 | CU8.2 CU7.2 | CU8.2 CU1.2 | LDPW5.C v64.77,38.1 64.77,39.37
  pour Top: 0,73.66 0,0 99.06,0 99.06,73.66
GREEN
  Bottom 0.356: 69.63,23.45 70.48,22.6 RL4.1 | IC3.9 69.56,23.52
  Bottom 0.406: 69.56,23.52 69.63,23.45
HWB
  Bottom 0.406: 32U4.33 41.27,56.6 41.27,57.78 RK7.2
I2C+5V
  Bottom 0.406: D7.A 80.64,59.05 87,59.05 87,59.96 J2.+5V
I2C+12V
  Bottom 1.27: J2.+12V 83.82,55.88 83.82,50.8 79.78,50.8 IC2.1
ISP+5V  (via drill 0.3, 0.35)
  Top 0.406: v31.75,40.64 32.38,40.64 v32.38,35.88
  Bottom 0.406: CON_ISP.5V 29.84,40.64 v31.75,40.64 | CON_ISP1.VCC 7.96,48.26 6.82,49.4 5.88,49.4 5.21,48.73 5.21,41.02 13.21,33.66 v32.38,33.66 v32.38,35.88
  Bottom 1.27: CON_ISP1.VCC 14.61,48.26 14.61,71.75 83.82,71.75 D8.A
MEM_SEL
  Bottom 0.406: R7.1 29.84,31.75 30.48,31.11 30.48,22.86 28.57,20.95 27.06,20.95 U$13.CE
MISO  (via drill 0.35)
  Top 0.356: v65.41,22.23 59.75,22.23 59.49,21.96 58.86,21.96 58.71,22.11 38.73,22.11
  Top 0.406: 38.73,22.11 26.14,22.11 v25.4,22.86 25.4,34.04 v25.97,34.61
  Bottom 0.356: IC3.11 v65.41,22.23
  Bottom 0.406: CON_ISP.MISO 29.84,36.83 30.48,36.83 | 30.48,36.83 32.83,36.83 32U4.11 | 30.48,36.83 30.48,34.61 v25.97,34.61 20,34.61 9.53,46.99 7.62,46.99 CON_ISP1.MISO | v25.4,22.86 U$13.SO
MOSI  (via drill 0.3, 0.35)
  Top 0.406: v33.66,41.77 v28.57,41.77 22.23,41.77 v22.23,41.74 | v12.7,46.99 12.7,50.16 12.06,50.8 CON_ISP1.MOSI | v59.69,23.5 59.05,24.13 v27.94,24.13
  Bottom 0.406: CON_ISP.MOSI v28.57,41.77 | 32U4.10 33.63,41.8 v33.66,41.77 33.66,34.29 33.14,33.78 33.14,33.16 32.88,32.9 26.61,32.9 26.55,32.95 21.2,32.95 20.49,32.24 20.49,29.69 RK4.1 19.92,28.65 U$13.SI 22.86,24.13 v27.94,24.13 | v22.23,41.74 16.05,41.74 15.24,42.55 15.24,45.09 13.97,46.35 13.34,46.35 v12.7,46.99 | IC3.5 60.31,22.88 v59.69,23.5
N$1
  Bottom 0.406: C13.2 36.83,40.77 32U4.6
N$2
  Top 0.406: U$11.3 22.61,61.59 R6.2
  Bottom 0.406: U$11.3
N$3
  Bottom 0.406: R9.2 48.26,29.21 48.26,34.29 L1.A
N$4
  Bottom 0.406: LED1.C R1.1
N$5
  Bottom 0.406: R4.2 R1.2 73.19,60.96 73.19,65.09 U1.1
N$6
  Bottom 0.406: U1.5 76.52,65.09 R5.1
N$7
  Bottom 0.406: R4.1 LED2.A
N$8
  Bottom 0.406: R2.2 46.99,26.67 46.99,31.11 L2.A
N$9
  Bottom 0.406: R10.2 RT3.2 89.53,20.32 86.36,23.5 83.61,23.5 X3.4
N$11
  Bottom 0.406: U$11.15 53.91,68.84 55.13,70.06 56.13,70.06 56.84,69.34 56.84,68.34 55.56,67.05 220.2
N$12
  Bottom 0.406: R13.2 64.77,34.61 LDPW5.A
N$15
  Bottom 0.406: C2.1 76.86,69.85 | 75.16,44.62 Q1.1 | LED1.A 60.33,60.96 60.33,59.05 74.3,59.05 | 75.16,50.8 IC2.3 75.49,50.88 75.56,50.8
  Bottom 1.27: D4.C D8.C 83.82,67.63 R3.2 | 75.16,44.62 D5.A | 75.16,44.62 75.56,44.62 75.56,50.8 | R3.2 D7.C 78.74,63.73 78.74,59.69 74.3,59.69 74.3,59.05 74.3,50.8 75.16,50.8 | 76.86,69.85 U1.4 80.64,66.99 R3.2
N$17  (via drill 0.35)
  Top 0.406: v55.24,34.29 71.75,34.29 72.39,34.92 AMP.1
  Bottom 0.406: R8.2 54.29,39.98 54.63,39.64 54.63,34.9 v55.24,34.29
  Bottom 1.27: Q1.2 72.16,44.62 D5.C | D5.C 72.39,41.27 | AMP.1 72.39,41.05 D5.C
N$19
  Bottom 0.406: U$6.5 CU4.2
N$20
  Bottom 0.406: U$6.3 33.97,29.4 33.27,28.7 33.27,27.32 33.34,27.25 CU4.1
N$23
  Bottom 0.406: RK1.2 29.21,26.04 28.57,25.4 24.77,25.4 24.13,26.04 U$13.SCK
N$42
  Bottom 0.406: 32U4.17 27.94,50.8 27.94,53.34 25.4,53.34 X2.P$2 22.23,53.37 RXT.2 19.68,51.75 CX1.2
RED
  Bottom 0.356: RL2.2 73.03,21.55 70.45,24.13 | IC3.8 70.4,24.18
  Bottom 0.406: 70.4,24.18 70.45,24.13
RESET  (via drill 0.3)
  Top 0.406: v16.51,56.52 6.35,56.52 CON_ISP1.RESET
  Bottom 0.406: 32U4.13 29.54,47.6 29.54,42.87 RK3.1 | CON_ISP.RESET 27.3,36.2 24.13,36.2 RK3.1 | RK3.1 16.51,42.87 v16.51,56.52
RX  (via drill 0.3)
  Top 0.406: v34.1,53.21 34.62,53.21 34.62,40.5 51.13,40.5 51.13,27.94 75.56,27.94 75.56,12.7 U$1.B
  Bottom 0.406: 32U4.20 v34.1,53.2 v34.1,53.21
SCK  (via drill 0.35)
  Top 0.406: v59.17,22.72 59.17,22.74 58.74,23.18 26.99,23.18 26.67,23.5 26.67,28.57 | 26.67,28.57 28.57,30.48 v29.21,30.48 | v11.03,46.59 11.03,48.03 9.53,49.53 7.62,49.53 CON_ISP1.SCK | 26.67,28.57 26.67,30.01 26.52,30.16 26.52,31.9 26.67,32.04 26.67,33.02 27.69,34.04 v27.69,35.47 28.23,34.92 v34.44,34.92
  Bottom 0.356: IC3.4 59.67,22.23 v59.17,22.72
  Bottom 0.406: v29.21,30.48 RK1.1 | CON_ISP.SCK 28.57,36.2 27.94,35.56 27.77,35.56 | 27.77,35.56 27.6,35.56 27.58,35.54 20.18,35.54 v11.03,46.59 | 27.77,35.56 v27.69,35.47 | 32U4.9 v34.43,34.93 v34.44,34.92
SCL  (via drill 0.3)
  Top 0.406: v39.73,51.6 39.73,57.15 87,57.15 87,53.98 91.68,53.98 J2.SCL
  Bottom 0.406: v39.73,51.6 39.73,51.44 32U4.18
SDA  (via drill 0.3)
  Top 0.406: J2.SDA 38.76,57.92 v38.76,52.7
  Bottom 0.406: v38.76,52.7 38.79,52.4 32U4.19
TX  (via drill 0.3)
  Top 0.406: v35.42,53.98 35.42,41.27 52.07,41.27 52.07,28.91 77.47,28.91 U$1.A
  Bottom 0.406: 32U4.21 v35.42,53.98
USB_N  (via drill 0.3)
  Top 0.406: v55.24,32.03 v60.95,32.03
  Bottom 0.406: 32U4.3 39.29,45 39.29,38.1 52.7,38.1 52.7,32.03 v55.24,32.03 | v60.95,32.03 78.42,32.03 78.42,45.72 RUSB1.1
USB_P  (via drill 0.3)
  Top 0.406: v55.24,31.04 v60.95,31.04
  Bottom 0.406: 32U4.4 38.47,45 38.47,36.83 | v60.95,31.04 79.38,31.04 79.38,43.18 RUSB2.1 | v55.24,31.04 51.44,31.04 51.44,36.83 38.47,36.83 | 38.47,36.83 38.47,36.75
USBC_N
  Bottom 0.406: X4.2 87.3,43.98 87.3,45.72 RUSB1.2
USBC_P
  Bottom 0.406: X4.3 RUSB2.2
V-
  Bottom 0.406: U$6.1 32.32,30.66 32.32,31.1 33.24,32.02 37.01,32.02 38.87,30.16 CU2.1 40.33,31.11 L2.K L1.K
VBAT1
  Bottom 0.406: C3.1 U1.3
  Bottom 1.27: 71.12,66.67 C3.1 71.12,69.85 63.68,69.85 | Q1.3 73.66,46.81 72.18,46.81 72.18,57.15 58.42,57.15 58.42,69.85 63.68,69.85 | JP1.1 63.5,69.67 63.68,69.85
VCC  (via drill 0.35, 0.7)
  Top 0.406: U$11.2 19.7,68.84 18.48,70.06 16.58,70.06 16.32,69.79 16.32,65.84 15.88,65.41 7.4,65.41 4.03,62.03 4.03,61.16 4.64,60.54 6.44,60.54 R6.3 | v26.04,17.14 26.04,12.21 25.89,12.06 | v21.59,30.48 19.72,30.48 19.68,30.52 | v27.3,30.48 27.3,31.75 27.94,32.38 33.39,32.38 v35.09,30.68
  Top 1.27: v70.01,54.93 81.44,54.93 81.28,27.81 | 81.28,27.81 v81.28,27.3 | v19.68,44.45 19.68,30.52 19.68,12.06 25.89,12.06 U$7.VDD | J3.+5V 11.7,27.67 12.7,26.67 12.7,13.65 12.06,13.02 10.82,13.02 J1.+5V | X3.1 81.79,27.3 81.28,27.81
  Bottom 0.254: IC3.10 67.67,22.86
  Bottom 0.356: 63.91,20.93 IC3.2 | 63.91,20.93 IC3.13 IC3.12 | 67.67,22.86 66.04,22.86 65.41,23.5 | 65.41,24.29 65.41,23.5 | 65.41,24.29 65.41,24.77 66.32,25.68 81.28,25.68 | IC3.7 61.9,24.29 65.41,24.29 | 65.41,23.5 65.41,23.29 64.65,22.54 64.65,21.67 63.91,20.93
  Bottom 0.406: C12.2 42.55,44.45 42.55,46.8 32U4.44 40.98,46.8 40.8,53.98 | 32U4.14 28.74,48.4 28.74,44.77 RK3.2 | 40.8,53.98 40.8,54.8 32U4.34 | 33.66,56.6 32U4.24 | 33.66,56.6 33.66,54.77 36.22,54.77 36.22,53.98 40.8,53.98 | 220.1 55.56,54.98 53.18,54.98 | U$11.2 20.07,66.92 23.5,63.5 28.71,63.5 28.73,63.48 33.04,63.48 33.66,62.87 33.66,56.6 | CU3.1 35.61,30.16 v35.09,30.68 34.41,31.36 33.53,31.36 33.27,31.1 33.27,30.66 U$6.2 | v26.04,17.14 C5.2 24.13,17.46 U$13.WP 24.13,22.23 23.52,22.84 23.22,22.84 23.2,22.86 22.23,22.86 19.68,25.4 RK4.2 | RT3.1 89.53,17.14 88.27,15.88 81.59,15.88 81.28,15.56 | v21.59,30.48 24.77,30.48 25.4,29.84 U$13.RST/HOLD U$13.VDD 26.67,29.84 v27.3,30.48 | 59.69,1.99 50.08,1.59 | VOLT.1 73.12,1.59 | U$12.8 34.63,12.4 34.29,12.06 U$7.VDD
  Bottom 0.813: IC1.3 62.23,45.16 | 61.72,54.98 53.18,54.98 40.98,54.98 40.98,46.8
  Bottom 1.27: R13.1 62.23,39.37 CU1.1 CU8.1 62.46,41.91 IC1.3 61.72,45.16 61.72,54.98 69.85,54.98 v70.01,54.93 | v81.28,27.3 81.28,25.68 81.28,15.56 81.44,1.59 73.12,1.59 50.08,1.59 28.57,1.59 28.57,5.72 | 28.57,5.72 28.57,12.06 U$7.VDD 11.43,11.91 10.55,12.62 J1.+5V | v19.68,44.45 24.13,44.45 RK3.2 | RT2.1 28.58,5.71 28.57,5.72
VDD
  Bottom 0.406: 67.08,44.62 IC1.1 67.31,45.16 | CU7.1 69.22,41.91
  Bottom 1.27: 67.08,44.62 68.89,44.62 CU7.1 68.89,34.92 74.93,34.92 AMP.2
VUSB  (via drill 0.3)
  Top 0.406: v55.24,33.02 v60.95,33.02
  Bottom 0.406: 40.01,45 40.01,46.99 36.03,46.99 32U4.7 | 32U4.2 40.01,45 | 40.01,45 40.01,39.37 53.98,39.37 53.98,33.02 v55.24,33.02 | v60.95,33.02 77.47,33.02 77.47,47.62 88.27,47.62 | 88.27,47.62 88.27,44.78 X4.1 | 88.27,47.62 88.27,49.53 97.16,49.53 97.16,62.53 85.72,62.53 85.72,60.73 D4.A
XTAL1
  Bottom 0.406: RXT.1 22.23,48.26 25.4,48.26 | 25.4,48.26 X2.P$1 | 25.4,48.26 27.94,48.26 27.94,50 32U4.16 | 21.59,49.66 RXT.1 | CX2.2 19.68,49.85 RXT.1

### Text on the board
tNames: 1 | BLK | D11 | EC11E / Encoder | 5V
bNames: Bio4_LCD_v1.1
tValues: Simple spectrophotometer PRO v.1.0.0
bValues: Simple spectrophotometer PRO v1.0.0

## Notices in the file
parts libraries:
lpatiny: ©2009 ROFA.cz - modified and updated by Robert Darlington ‹rdarlington@gmail.com›
microbuilder: This work is placed in the public domain, and may be freely used for commercial and non-commercial work with the following conditions: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
